| IBIS file abc.ibs created by s2ibis2 version 1.2
| North Carolina State University Electronics Research Laboratory  1995
[IBIS ver]   2.1
[File name]   70t653m.ibs
[File Rev]   1.0
|1.0 : Original Version (Changed C_comp values from 9M Async) - Sunil Kashyap
[Date]   01/20/2004
[Source]   Integrated Device Technology, Inc.
[Notes]   1.Temperatures: typ=25C, min=100C, max=0C 2.RRmp rates based
   on 50 ohm load.
[Disclaimer] Integrated Device Technology, Inc. ("IDT") hereby grants the
   user of this IBIS model a non-exclusive, nontransferable
   license to use this IBIS model under the following terms. The
   user is granted this license only to use the IBIS model and is
   not granted rights to sell, copy (except as needed to run the
   IBIS model), rent, lease or sub-license the IBIS model in
   whole or in part, or in modified form to anyone. The User may
   modify the IBIS model to suit its specific applications, but
   rights to derivative works and such modifications shall belong
   to IDT. This IBIS model is provided on an AS IS" basis and IDT
   makes absolutely no warranty with respect to the information
   contained herein. IDT DISCLAIMS AND CUSTOMER WAIVES ALL
   WARRANTIES, EXPRESS AND IMPLIED, INCLUDING WARRANTIES OF
   MERCHANTABILITY AND FITNESS FOR A PARTICULAR PURPOSE. THE
   ENTIRE RISK AS TO QUALITY AND PERFORMANCE IS WITH THE USER
   ACCORDINGLY, IN NO EVENT SHALL IDT BE LIABLE FOR ANY DIRECT OR
   INDIRECT DAMAGES, WHETHER IN CONTRACT OR TORT, INCLUDING ANY
   LOST PROFITS OR OTHER INCIDENTAL, CONSEQUENTIAL, EXEMPLARY, OR
   PUNITIVE DAMAGES ARISING OUT OF THE USE OR APPLICATION OF THE
   IBIS model. Further, IDT reserves the right to make changes
   without notice to any product herein to improve reliability,
   function, or design. IDT does not convey any license under
   patent rights or any other intellectual property rights,
   including those of third parties. IDT is not obligated to
   provide maintenance or support for the licensed IBIS model.
[Copyright]   Copyright 2001, Integrated Device Technology, Inc. all rights
   reserved
|   Component idt70t6xx_256BC
[Component]   idt70t6xx_256BC
[Manufacturer]   Integrated Device Technology
[Package]
| variable   typ   min   max
R_pkg   0.16200   0.13000   0.19400
L_pkg   4.82000nH   3.56000nH   6.07000nH
C_pkg   1.47000pF   1.28000pF   1.66000pF
| NOTE:
| The model_name inpad25, inpadzz25, inpadbs25, and iopad25 work for
| both 3.3v and 2.5v vddq.  When vddq is 3.3v, the model names are
| inpad33, inpadzz33, inpadbs33, and iopad33.  When vddq is 2.5v,
| the model names will be inpad25, inpadzz25, inpadbs25,and iopad25.
[Pin]  signal_name   model_name   R_pin   L_pin   C_pin
C2   io19l   iopad25
D2   io19r   iopad25
D3   io20l   iopad25
D1   io20r   iopad25
D5   vddql   POWER
E7   vss   GND
E2   io21l   iopad25
E1   io21r   iopad25
E3   io22l   iopad25
F2   io22r   iopad25
D7   vddqr   POWER
E8   vss   GND
F1   io23l   iopad25
F3   io23r   iopad25
G2   io24l   iopad25
G1   io24r   iopad25
D6   vddql   POWER
F6   vss   GND
G3   io25l   iopad25
H2   io25r   iopad25
H1   io26l   iopad25
H3   io26r   iopad25
G4   vddqr   POWER
G5   vss   GND
D4   vdd   POWER
E5   vdd   POWER
G6   vss   GND
G7   vss   GND
J4   vddql   POWER
J5   zzr   inpadzz25
J3   io27r   iopad25
J1   io27l   iopad25
J2   io28r   iopad25
K3   io28l   iopad25
M4   vddqr   POWER
K5   vss   GND
K1   io29r   iopad25
K2   io29l   iopad25
L3   io30r   iopad25
L1   io30l   iopad25
N7   vddql   POWER
M7   vss   GND
L2   io31r   iopad25
M3   io31l   iopad25
M1   io32r   iopad25
M2   io32l   iopad25
N5   vddqr   POWER
L6   vss   GND
N3   io33r   iopad25
N1   io33l   iopad25
N2   io34r   iopad25
P2   io34l   iopad25
K7   vss   GND
K4   vddql   POWER
P1   io35r   iopad25
R1   io35l   iopad25
L5   vdd   POWER
P3   tms   inpadbs25
T2   tck   inpadbs25
R3   trstb   inpadbs25
R4   a18r   inpad25
T4   a17r   inpad25
P4   a16r   inpad25
R5   a15r   inpad25
T5   a14r   inpad25
P5   a13r   inpad25
R6   a12r   inpad25
T6   a11r   inpad25
P6   a10r   inpad25
R7   a9r   inpad25
T7   a8r   inpad25
P7   a7r   inpad25
R8   be3rb   inpad25
T8   be2rb   inpad25
P8   be1rb   inpad25
P9   be0rb   inpad25
T9   ce1r   inpad25
R9   ce0r   inpad25
M5   vdd   POWER
M6   vdd   POWER
K6   vss   GND
L7   vss   GND
P10   semrb   inpad25
T10   oerb   inpad25
R10   rwrb   inpad25
P11   busyrb   iopad25
T11   intrb   iopad25
R11   msrb   inpad25
P12   a6r   inpad25
T12   a5r   inpad25
R12   a4r   inpad25
P13   a3r   inpad25
T13   a2r   inpad25
R13   a1r   inpad25
T14   a0r   inpad25
N13   vdd   POWER
M8   vss   GND
M9   vss   GND
R14   optr   inpad25
P14   io0l   iopad25
P15   io0r   iopad25
N12   vddql   POWER
M10   vss   GND
P16   io1l   iopad25
N15   io1r   iopad25
N14   io2l   iopad25
N16   io2r   iopad25
N10   vddqr   POWER
L9   vss   GND
M15   io3l   iopad25
M14   io3r   iopad25
M16   io4l   iopad25
L15   io4r   iopad25
N8   vddql   POWER
L8   vss   GND
L14   io5l   iopad25
L16   io5r   iopad25
K15   io6l   iopad25
K14   io6r   iopad25
N6   vddqr   POWER
K8   vss   GND
K16   io7l   iopad25
J15   io7r   iopad25
J16   io8l   iopad25
J14   io8r   iopad25
N11   vddql   POWER
L11   vss   GND
K11   vss   GND
K12   vss   GND
M11   vdd   POWER
M12   vdd   POWER
N9   vddqr   POWER
L10   vss   GND
H14   io9r   iopad25
H15   io9l   iopad25
H16   io10r   iopad25
G14   io10l   iopad25
M13   vddql   POWER
K10   vss   GND
G16   io11r   iopad25
G15   io11l   iopad25
F14   io12r   iopad25
F16   io12l   iopad25
K13   vddqr   POWER
K9   vss   GND
F15   io13r   iopad25
E14   io13l   iopad25
E16   io14r   iopad25
E15   io14l   iopad25
L13   vddql   POWER
J12   zzl   inpadzz25
D14   io15r   iopad25
D15   io15l   iopad25
D16   io16r   iopad25
C16   io16l   iopad25
J11   vss   GND
J13   vddqr   POWER
C15   io17r   iopad25
B15   io17l   iopad25
C14   optl   inpad25
H12   vss   GND
L12   vdd   POWER
D13   vdd   POWER
A14   a0l   inpad25
B13   a1l   inpad25
A13   a2l   inpad25
C13   a3l   inpad25
B12   a4l   inpad25
A12   a5l   inpad25
C12   a6l   inpad25
A11   intlb   iopad25
C11   busylb   iopad25
B10   rwlb   inpad25
A10   oelb   inpad25
C10   semlb   inpad25
G11   vss   GND
G12   vss   GND
E12   vdd   POWER
F12   vdd   POWER
B9   ce0lb   inpad25
A9   ce1l   inpad25
C9   be0lb   inpad25
C8   be1lb   inpad25
A8   be2lb   inpad25
B8   be3lb   inpad25
C7   a7l   inpad25
A7   a8l   inpad25
B7   a9l   inpad25
C6   a10l   inpad25
A6   a11l   inpad25
B6   a12l   inpad25
C5   a13l   inpad25
A5   a14l   inpad25
B5   a15l   inpad25
C4   a16l   inpad25
A4   a17l   inpad25
B4   a18l   inpad25
B3   tdo   iopad25
A2   tdi   inpadbs25
E6   vdd   POWER
C3   test/vss   GND
B1   io18l   iopad25
C1   io18r   iopad25
H4   vddqr   POWER
H5   vss   GND
E4   vddql   POWER
F7   vss   GND
F4   vddql   POWER
H7   vss   GND
D9   vddql   POWER
E9   vss   GND
D10   vddql   POWER
E10   vss   GND
G13   vddql   POWER
F11   vss   GND
H13   vddql   POWER
H11   vss   GND
L4   vddqr   POWER
J6   vss   GND
E13   vddqr   POWER
F10   vss   GND
F13   vddqr   POWER
G10   vss   GND
D11   vddqr   POWER
F8   vss   GND
D12   vddqr   POWER
F9   vss   GND
D8   vddqr   POWER
G8   vss   GND
E11   vdd   POWER
G9   vss   GND
H6   vss   GND
H8   vss   GND
H9   vss   GND
H10   vss   GND
J7   vss   GND
J8   vss   GND
J9   vss   GND
J10   vss   GND
|in   in   dummy_model
|oe   oe   dummy_model
| needed to give pads seperate POWER supply
[Pin Mapping] pulldown_ref   pullup_ref
C2   vss   vddql
D2   vss   vddqr
D3   vss   vddql
D1   vss   vddqr
D5   nc   vddql
E7   vss   nc
E2   vss   vddql
E1   vss   vddqr
E3   vss   vddql
F2   vss   vddqr
D7   nc   vddqr
E8   vss   nc
F1   vss   vddql
F3   vss   vddqr
G2   vss   vddql
G1   vss   vddqr
D6   nc   vddql
F6   vss   nc
G3   vss   vddql
H2   vss   vddqr
H1   vss   vddql
H3   vss   vddqr
G4   nc   vddqr
G5   vss   nc
D4   nc   vdd
E5   nc   vdd
G6   vss   nc
G7   vss   nc
J4   nc   vddql
J5   vss   nc
J3   vss   vddqr
J1   vss   vddql
J2   vss   vddqr
K3   vss   vddql
M4   nc   vddqr
K5   vss   nc
K1   vss   vddqr
K2   vss   vddql
L3   vss   vddqr
L1   vss   vddql
N7   nc   vddql
M7   vss   nc
L2   vss   vddqr
M3   vss   vddql
M1   vss   vddqr
M2   vss   vddql
N5   nc   vddqr
L6   vss   nc
N3   vss   vddqr
N1   vss   vddql
N2   vss   vddqr
P2   vss   vddql
K7   vss   nc
K4   nc   vddql
P1   vss   vddqr
R1   vss   vddql
L5   nc   vdd
P3   vss   vdd
T2   vss   vdd
R3   vss   vdd
R4   vss   vdd
T4   vss   vdd
P4   vss   vdd
R5   vss   vdd
T5   vss   vdd
P5   vss   vdd
R6   vss   vdd
T6   vss   vdd
P6   vss   vdd
R7   vss   vdd
T7   vss   vdd
P7   vss   vdd
R8   vss   vdd
T8   vss   vdd
P8   vss   vdd
P9   vss   vdd
T9   vss   vdd
R9   vss   vdd
M5   nc   vdd
M6   nc   vdd
K6   vss   nc
L7   vss   nc
P10   vss   vdd
T10   vss   vdd
R10   vss   vdd
P11   vss   vdd
T11   vss   vdd
R11   vss   vdd
P12   vss   vdd
T12   vss   vdd
R12   vss   vdd
P13   vss   vdd
T13   vss   vdd
R13   vss   vdd
T14   vss   vdd
N13   nc   vdd
M8   vss   nc
M9   vss   nc
R14   vss   vdd
P14   vss   vddql
P15   vss   vddqr
N12   nc   vddql
M10   vss   nc
P16   vss   vddql
N15   vss   vddqr
N14   vss   vddql
N16   vss   vddqr
N10   nc   vddqr
L9   vss   nc
M15   vss   vddql
M14   vss   vddqr
M16   vss   vddql
L15   vss   vddqr
N8   nc   vddql
L8   vss   nc
L14   vss   vddql
L16   vss   vddqr
K15   vss   vddql
K14   vss   vddqr
N6   nc   vddqr
K8   vss   nc
K16   vss   vddql
J15   vss   vddqr
J16   vss   vddql
J14   vss   vddqr
N11   nc   vddql
L11   vss   nc
K11   vss   nc
K12   vss   nc
M11   nc   vdd
M12   nc   vdd
N9   nc   vddqr
L10   vss   nc
H14   vss   vddqr
H15   vss   vddql
H16   vss   vddqr
G14   vss   vddql
M13   nc   vddql
K10   vss   nc
G16   vss   vddqr
G15   vss   vddql
F14   vss   vddqr
F16   vss   vddql
K13   nc   vddqr
K9   vss   nc
F15   vss   vddqr
E14   vss   vddql
E16   vss   vddqr
E15   vss   vddql
L13   nc   vddql
J12   vss   nc
D14   vss   vddqr
D15   vss   vddql
D16   vss   vddqr
C16   vss   vddql
J11   vss   nc
J13   nc   vddqr
C15   vss   vddqr
B15   vss   vddql
C14   vss   vdd
H12   vss   nc
L12   nc   vdd
D13   nc   vdd
A14   vss   vdd
B13   vss   vdd
A13   vss   vdd
C13   vss   vdd
B12   vss   vdd
A12   vss   vdd
C12   vss   vdd
A11   vss   vdd
C11   vss   vdd
B10   vss   vdd
A10   vss   vdd
C10   vss   vdd
G11   vss   nc
G12   vss   nc
E12   nc   vdd
F12   nc   vdd
B9   vss   vdd
A9   vss   vdd
C9   vss   vdd
C8   vss   vdd
A8   vss   vdd
B8   vss   vdd
C7   vss   vdd
A7   vss   vdd
B7   vss   vdd
C6   vss   vdd
A6   vss   vdd
B6   vss   vdd
C5   vss   vdd
A5   vss   vdd
B5   vss   vdd
C4   vss   vdd
A4   vss   vdd
B4   vss   vdd
B3   vss   vdd
A2   vss   vdd
E6   nc   vdd
C3   vss   nc
B1   vss   vddql
C1   vss   vddqr
H4   nc   vddqr
H5   vss   nc
E4   nc   vddql
F7   vss   nc
F4   nc   vddql
H7   vss   nc
D9   nc   vddql
E9   vss   nc
D10   nc   vddql
E10   vss   nc
G13   nc   vddql
F11   vss   nc
H13   nc   vddql
H11   vss   nc
L4   nc   vddqr
J6   vss   nc
E13   nc   vddqr
F10   vss   nc
F13   nc   vddqr
G10   vss   nc
D11   nc   vddqr
F8   vss   nc
D12   nc   vddqr
F9   vss   nc
D8   nc   vddqr
G8   vss   nc
E11   nc   vdd
G9   vss   nc
H6   vss   nc
H8   vss   nc
H9   vss   nc
H10   vss   nc
J7   vss   nc
J8   vss   nc
J9   vss   nc
J10   vss   nc
| Models and submodels in the file (8): inpad25 (Input), inpad33 (Input), inpadzz25 (Input), inpadzz33 (Input), inpadbs25 (Input), inpadbs33 (Input), iopad25 (I/O), iopad33 (I/O)
